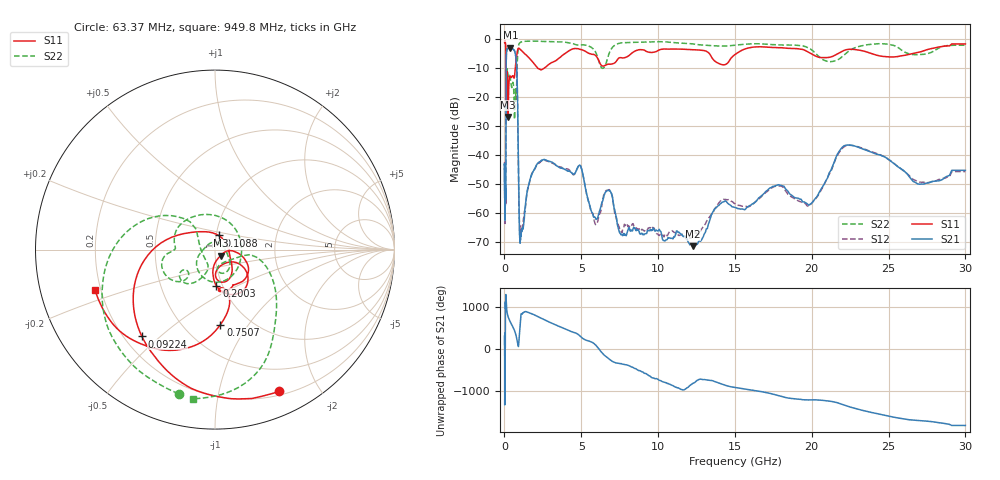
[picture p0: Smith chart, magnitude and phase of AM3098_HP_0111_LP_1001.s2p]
! Date/Time: Thu, Feb 28, 2019 8:38 AM
! Network Analyzer: Agilent Technologies E8364B Rev: A.07.50.67
! Sweep from 0.010 to 30.000 GHz, 1601 Points, Sweep Type: LOG
! Power Supply: 5.022 V, 0.002 A
# Hz S DB R 50
!freq MagS11 AngS11 MagS21 AngS21 MagS12 AngS12 MagS22 AngS22
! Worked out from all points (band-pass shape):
!   1601 points, 10 MHz to 30 GHz, reference 50 ohm
!   highest |S21| = -2.80 dB at 382 MHz (marker M1); lowest = -71.4 dB at 12.25 GHz (marker M2)
!   |S21| within 3 dB of the highest: 121.9 MHz to 735.8 MHz (613.9 MHz wide, 143 % of centre)
!   lowest |S11| = -26.8 dB at 238.7 MHz (marker M3), VSWR 1.10, Z = 53.1 - j3.59 ohm
!   |S11| at or under -10 dB: 102.2 MHz to 701.9 MHz (599.8 MHz wide, 149 % of centre); 2.187 GHz to 2.549 GHz (362.3 MHz wide, 15.3 % of centre)
!   |S22| runs from -27.6 to -0.5 dB; largest |S21 - S12| = 0.013
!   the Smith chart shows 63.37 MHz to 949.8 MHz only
!   S11 on the Smith chart (normalised r, x): 63.37 MHz: 0.24, -1.52; 92.24 MHz: 0.27, -0.44; 108.8 MHz: 1.03, +0.16; 200.3 MHz: 0.94, -0.39; 750.7 MHz: 0.74, -0.75; 949.8 MHz: 0.18, -0.16
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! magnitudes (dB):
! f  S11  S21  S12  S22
! 10 MHz  -0.3  -43.0  -42.9  -0.6
! 38.04 MHz  -0.5  -60.5  -59.9  -0.9
! 63.37 MHz  -1.2  -51.4  -57.2  -1.6
! 83.87 MHz  -2.4  -54.9  -55.9  -2.8
! 92.24 MHz  -4.0  -42.3  -41.6  -4.4
! 108.8 MHz  -21.8  -10.6  -10.6  -22.8
! 144.7 MHz  -19.9  -4.0  -3.9  -14.2
! 200.3 MHz  -13.9  -3.2  -3.2  -10.6
! 238.7 MHz  -26.8  -2.9  -2.9  -12.6
! 382 MHz  -12.8  -2.8  -2.8  -13.6
! 550.5 MHz  -12.5  -3.3  -3.3  -14.8
! 750.7 MHz  -7.6  -6.4  -6.4  -21.3
! 838.1 MHz  -4.1  -17.0  -17.0  -7.2
! 949.8 MHz  -3.0  -60.3  -59.0  -1.5
! 1.044 GHz  -3.5  -69.0  -66.9  -1.0
! 2.084 GHz  -9.4  -43.4  -43.4  -0.6
! 4.903 GHz  -3.4  -43.4  -43.2  -2.0
! 7.926 GHz  -6.1  -67.8  -64.3  -1.1
! 12.25 GHz  -3.5  -71.4  -68.0  -1.5
! 19.8 GHz  -4.5  -57.3  -57.6  -2.9
! 22.56 GHz  -3.4  -36.5  -36.6  -3.5
! 30 GHz  -1.5  -45.2  -45.6  -2.0
